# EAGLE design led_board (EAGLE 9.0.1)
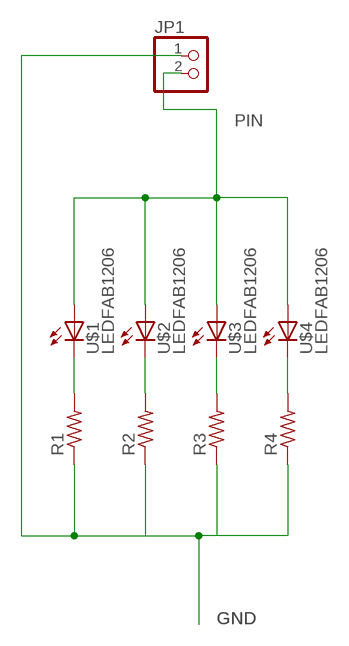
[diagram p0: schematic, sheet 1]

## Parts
JP1  PINHD-1X2  [1X02]
R1  RES-US1206FAB  [R1206FAB]
R2  RES-US1206FAB  [R1206FAB]
R3  RES-US1206FAB  [R1206FAB]
R4  RES-US1206FAB  [R1206FAB]
U$1  LEDFAB1206  [LED1206FAB]
U$2  LEDFAB1206  [LED1206FAB]
U$3  LEDFAB1206  [LED1206FAB]
U$4  LEDFAB1206  [LED1206FAB]

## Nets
GND: JP1.1 R1.1 R2.1 R3.1 R4.1
N$1: R1.2 U$1.2(C)
N$2: R2.2 U$2.2(C)
N$3: R3.2 U$3.2(C)
N$4: R4.2 U$4.2(C)
PIN: JP1.2 U$1.1(A) U$2.1(A) U$3.1(A) U$4.1(A)

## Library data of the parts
JP1 = pinhead:PINHD-1X2: PIN HEADER
R1-R4 = fab:RES-US: Resistor (US Symbol)
U$1-U$4 = fab:LED: LED

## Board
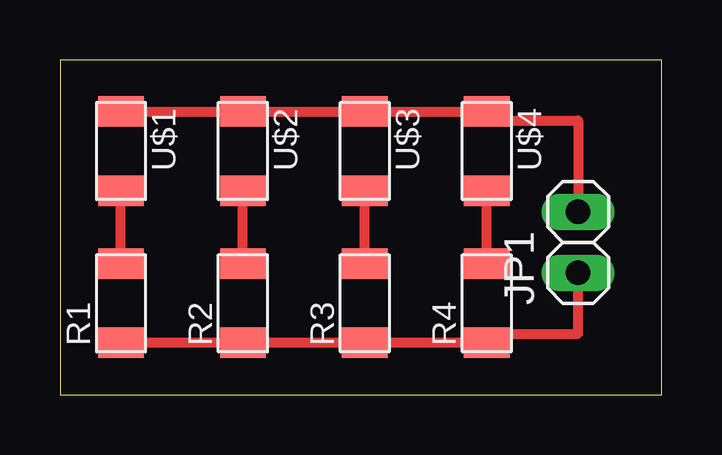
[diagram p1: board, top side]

Size 25.07 x 13.96 mm. Coordinates in mm from the lower left corner, seen from the top.
Outline: 0,0 25.07,0 25.07,13.96 0,13.96 0,0
Copper layers (1*16): Top 0.035mm / dielectric 1.5mm / Bottom 0.035mm
Design rules "default": minimum track width 6mil, minimum drill 0.35mm, track to track 6mil, track to pad 6mil, pad to pad 6mil, via to via 6mil, smd to smd 6mil, copper to edge 40mil, drill to drill 6mil, minimum pad ring 10mil, minimum via ring 8mil, stop-mask expansion 4mil, vias tented up to drill 0mil, thermal gap 10mil

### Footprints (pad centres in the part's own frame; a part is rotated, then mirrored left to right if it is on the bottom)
1X02 = drill 1.016 long: 1 -1.27,0; 2 1.27,0
R1206FAB = smd 1.27 x 1.905: 1 -1.651,0; 2 1.651,0
LED1206FAB = smd 1.27 x 1.905: 1 -1.651,0; 2 1.651,0

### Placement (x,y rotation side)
JP1  21.59,6.35 90 top
R1  2.54,3.81 90 top
R2  7.62,3.81 90 top
R3  12.7,3.81 90 top
R4  17.78,3.81 90 top
U$1  2.54,10.16 270 top
U$2  7.62,10.16 270 top
U$3  12.7,10.16 270 top
U$4  17.78,10.16 270 top

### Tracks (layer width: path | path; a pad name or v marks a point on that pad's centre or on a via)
GND
  Top 0.406: 2.16,2.54 arc-90 R1.1 R2.1 R3.1 R4.1 arc-90 18.16,2.54 21.59,2.54 JP1.1
N$1
  Top 0.406: R1.2 U$1.2
N$2
  Top 0.406: R2.2 U$2.2
N$3
  Top 0.406: R3.2 U$3.2
N$4
  Top 0.406: R4.2 U$4.2
PIN
  Top 0.406: U$1.1 U$2.1 U$3.1 U$4.1 arc90 18.16,11.43 21.59,11.43 JP1.2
